FUNCTION "PALLET IMP.LAT. SU USCIT" : VOID
TITLE =GESTIONE PALLET PROVENIENTE DA IMPIL. LATERALE SU BAIA USCITA
VERSION : 0.1
//KNOW_HOW_PROTECT

VAR_TEMP
  Error_block_move : INT ;
END_VAR
BEGIN
NETWORK
TITLE =

NETWORK
TITLE =Spostamento dati per pallet in transito tra ribaltat. e uscita
//- "Container Flag"
//- "Id TAG"
//- "FlagRibaltamento"
//- "Container_Id"
//- "Date LCB"
//- "Part Number"
//- "Quantity"
//- "Line Id"
//- "CIM"
//- "Colata Id"
//- "Material Of Test Flag"
//- "Lotto Id"
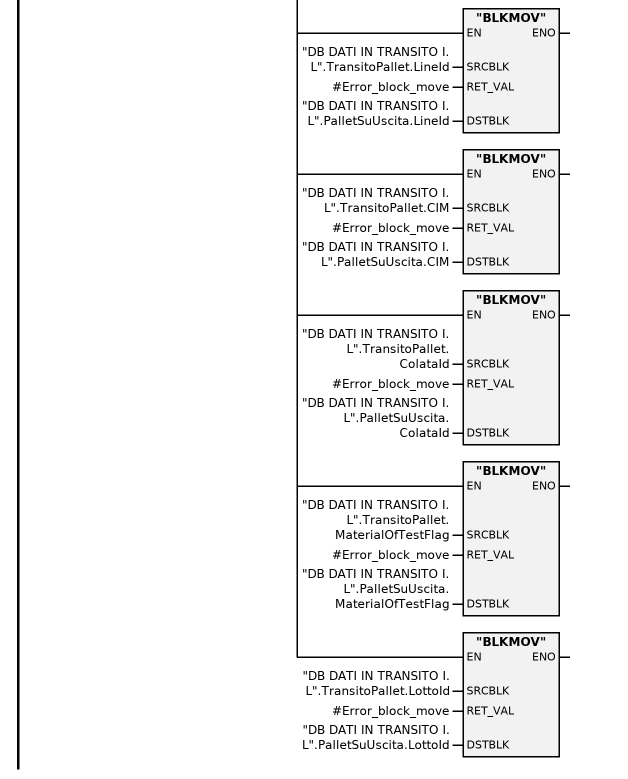
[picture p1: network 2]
      U     "M900.0";
      U     "DB SCAMBIO DATI PIANELLI".Pallet_I_L_su_uscita;
      FP    M    390.1;
      =     L      2.0;
      U     L      2.0;
      SPBNB _001;
      CALL "BLKMOV" (
           SRCBLK                   := "DB DATI IN TRANSITO I. L".TransitoPallet.ContainerFlag,
           RET_VAL                  := #Error_block_move,
           DSTBLK                   := "DB DATI IN TRANSITO I. L".PalletSuUscita.ContainerFlag);
_001: NOP   0;
      U     L      2.0;
      SPBNB _002;
      CALL "BLKMOV" (
           SRCBLK                   := "DB DATI IN TRANSITO I. L".TransitoPallet.ID_TAG,
           RET_VAL                  := #Error_block_move,
           DSTBLK                   := "DB DATI IN TRANSITO I. L".PalletSuUscita.ID_TAG);
_002: NOP   0;
      U     L      2.0;
      SPBNB _003;
      CALL "BLKMOV" (
           SRCBLK                   := "DB DATI IN TRANSITO I. L".TransitoPallet.FlagRibaltamento,
           RET_VAL                  := #Error_block_move,
           DSTBLK                   := "DB DATI IN TRANSITO I. L".PalletSuUscita.FlagRibaltamento);
_003: NOP   0;
      U     L      2.0;
      SPBNB _004;
      CALL "BLKMOV" (
           SRCBLK                   := "DB DATI IN TRANSITO I. L".TransitoPallet.Container_Id,
           RET_VAL                  := #Error_block_move,
           DSTBLK                   := "DB DATI IN TRANSITO I. L".PalletSuUscita.Container_Id);
_004: NOP   0;
      U     L      2.0;
      SPBNB _005;
      CALL "BLKMOV" (
           SRCBLK                   := "DB DATI IN TRANSITO I. L".TransitoPallet.DateLCB,
           RET_VAL                  := #Error_block_move,
           DSTBLK                   := "DB DATI IN TRANSITO I. L".PalletSuUscita.DateLCB);
_005: NOP   0;
      U     L      2.0;
      SPBNB _006;
      CALL "BLKMOV" (
           SRCBLK                   := "DB DATI IN TRANSITO I. L".TransitoPallet.PartNumber,
           RET_VAL                  := #Error_block_move,
           DSTBLK                   := "DB DATI IN TRANSITO I. L".PalletSuUscita.PartNumber);
_006: NOP   0;
      U     L      2.0;
      SPBNB _007;
      CALL "BLKMOV" (
           SRCBLK                   := "DB DATI IN TRANSITO I. L".TransitoPallet.Quantity,
           RET_VAL                  := #Error_block_move,
           DSTBLK                   := "DB DATI IN TRANSITO I. L".PalletSuUscita.Quantity);
_007: NOP   0;
      U     L      2.0;
      SPBNB _008;
      CALL "BLKMOV" (
           SRCBLK                   := "DB DATI IN TRANSITO I. L".TransitoPallet.LineId,
           RET_VAL                  := #Error_block_move,
           DSTBLK                   := "DB DATI IN TRANSITO I. L".PalletSuUscita.LineId);
_008: NOP   0;
      U     L      2.0;
      SPBNB _009;
      CALL "BLKMOV" (
           SRCBLK                   := "DB DATI IN TRANSITO I. L".TransitoPallet.CIM,
           RET_VAL                  := #Error_block_move,
           DSTBLK                   := "DB DATI IN TRANSITO I. L".PalletSuUscita.CIM);
_009: NOP   0;
      U     L      2.0;
      SPBNB _00a;
      CALL "BLKMOV" (
           SRCBLK                   := "DB DATI IN TRANSITO I. L".TransitoPallet.ColataId,
           RET_VAL                  := #Error_block_move,
           DSTBLK                   := "DB DATI IN TRANSITO I. L".PalletSuUscita.ColataId);
_00a: NOP   0;
      U     L      2.0;
      SPBNB _00b;
      CALL "BLKMOV" (
           SRCBLK                   := "DB DATI IN TRANSITO I. L".TransitoPallet.MaterialOfTestFlag,
           RET_VAL                  := #Error_block_move,
           DSTBLK                   := "DB DATI IN TRANSITO I. L".PalletSuUscita.MaterialOfTestFlag);
_00b: NOP   0;
      U     L      2.0;
      SPBNB _00c;
      CALL "BLKMOV" (
           SRCBLK                   := "DB DATI IN TRANSITO I. L".TransitoPallet.LottoId,
           RET_VAL                  := #Error_block_move,
           DSTBLK                   := "DB DATI IN TRANSITO I. L".PalletSuUscita.LottoId);
_00c: NOP   0;
NETWORK
TITLE =Lettura Pallet su baia di scarico
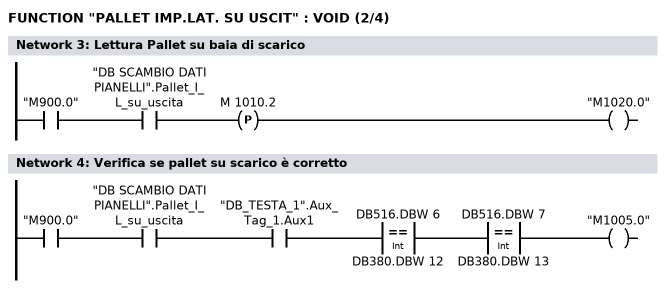
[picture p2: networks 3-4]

      U     "M900.0";
      U     "DB SCAMBIO DATI PIANELLI".Pallet_I_L_su_uscita;
      FP    M   1010.2;
      =     "M1020.0";
NETWORK
TITLE =Verifica se pallet su scarico è corretto

      U     "M900.0";
      U     "DB SCAMBIO DATI PIANELLI".Pallet_I_L_su_uscita;
      U     "DB_TESTA_1".Aux_Tag_1.Aux1;
      U(    ;
      L     DB516.DBW    6;
      L     DB380.DBW   12;
      ==I   ;
      )     ;
      U(    ;
      L     DB516.DBW    7;
      L     DB380.DBW   13;
      ==I   ;
      )     ;
      =     "M1005.0";
NETWORK
TITLE =Se pallet è corretto e ribaltato, aggiorno TAG
//- "Container Flag"
//- "Id TAG"
//- "FlagRibaltamento"
//- "Container_Id"
//- "Date LCB"
//- "Part Number"
//- "Quantity"
//- "Line Id"
//- "CIM"
//- "Colata Id"
//- "Material Of Test Flag"
//- "Lotto Id"
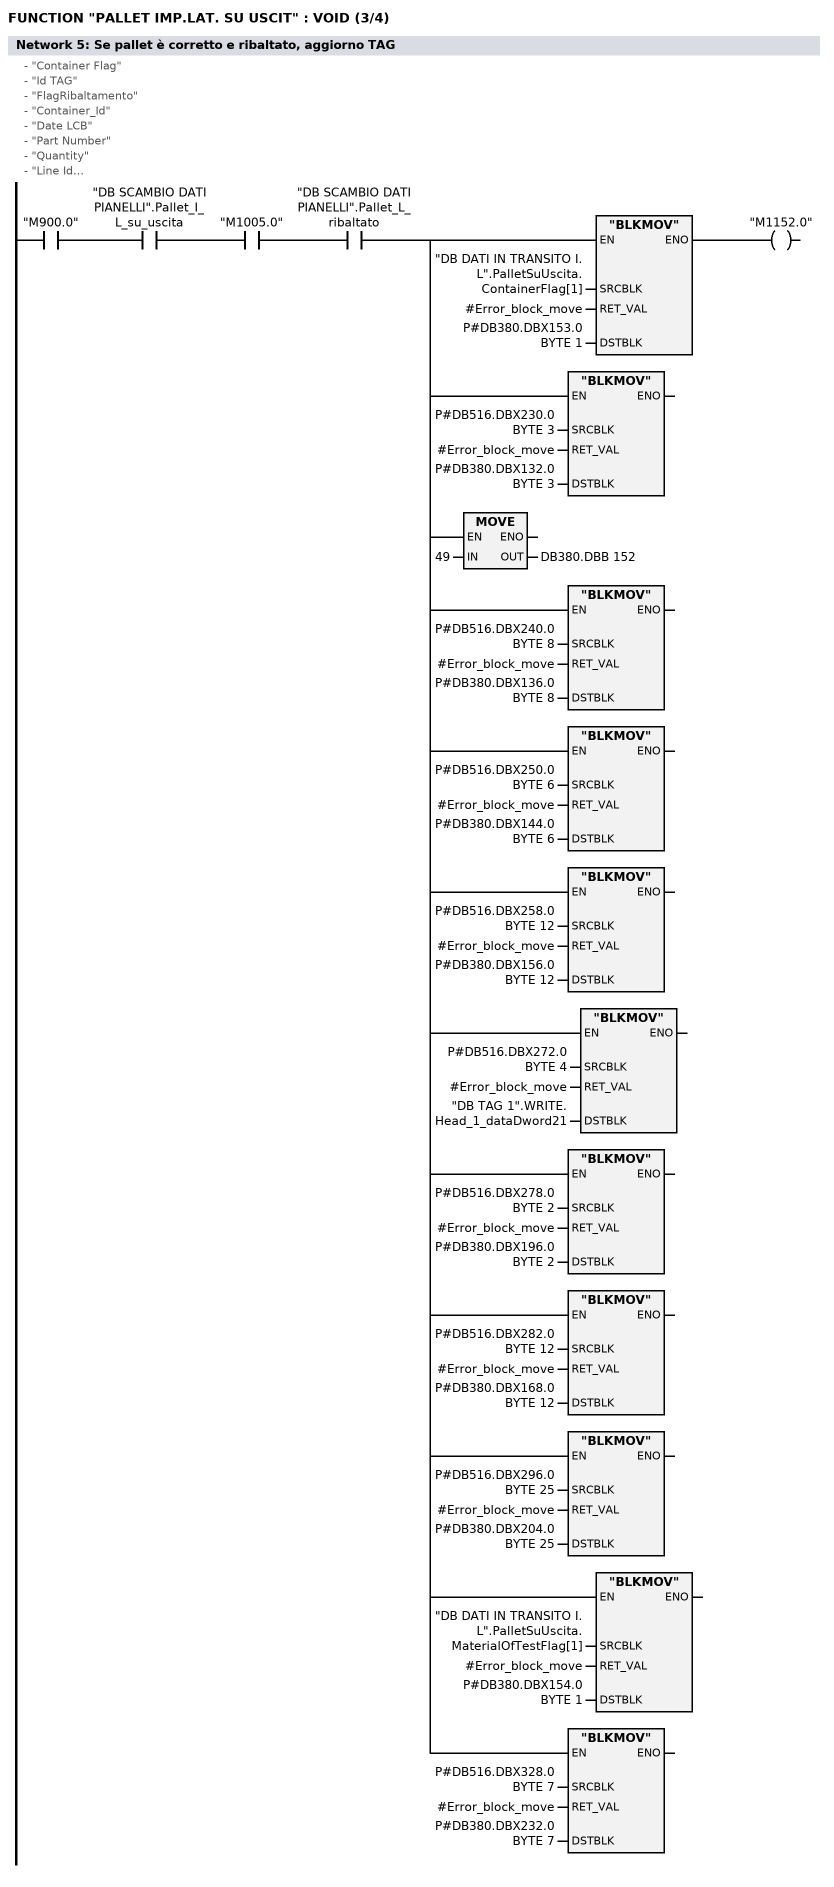
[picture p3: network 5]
      U     "M900.0";
      U     "DB SCAMBIO DATI PIANELLI".Pallet_I_L_su_uscita;
      U     "M1005.0";
      U     "DB SCAMBIO DATI PIANELLI".Pallet_L_ribaltato;
      =     L      2.0;
      U     L      2.0;
      SPBNB _00d;
      CALL "BLKMOV" (
           SRCBLK                   := "DB DATI IN TRANSITO I. L".PalletSuUscita.ContainerFlag[1],
           RET_VAL                  := #Error_block_move,
           DSTBLK                   := P#DB380.DBX153.0 BYTE 1);
_00d: U     BIE;
      =     "M1152.0";
      U     L      2.0;
      SPBNB _00e;
      CALL "BLKMOV" (
           SRCBLK                   := P#DB516.DBX230.0 BYTE 3,
           RET_VAL                  := #Error_block_move,
           DSTBLK                   := P#DB380.DBX132.0 BYTE 3);
_00e: NOP   0;
      U     L      2.0;
      SPBNB _00f;
      L     49;
      T     DB380.DBB  152;
_00f: NOP   0;
      U     L      2.0;
      SPBNB _010;
      CALL "BLKMOV" (
           SRCBLK                   := P#DB516.DBX240.0 BYTE 8,
           RET_VAL                  := #Error_block_move,
           DSTBLK                   := P#DB380.DBX136.0 BYTE 8);
_010: NOP   0;
      U     L      2.0;
      SPBNB _011;
      CALL "BLKMOV" (
           SRCBLK                   := P#DB516.DBX250.0 BYTE 6,
           RET_VAL                  := #Error_block_move,
           DSTBLK                   := P#DB380.DBX144.0 BYTE 6);
_011: NOP   0;
      U     L      2.0;
      SPBNB _012;
      CALL "BLKMOV" (
           SRCBLK                   := P#DB516.DBX258.0 BYTE 12,
           RET_VAL                  := #Error_block_move,
           DSTBLK                   := P#DB380.DBX156.0 BYTE 12);
_012: NOP   0;
      U     L      2.0;
      SPBNB _013;
      CALL "BLKMOV" (
           SRCBLK                   := P#DB516.DBX272.0 BYTE 4,
           RET_VAL                  := #Error_block_move,
           DSTBLK                   := "DB TAG 1".WRITE.Head_1_dataDword21);
_013: NOP   0;
      U     L      2.0;
      SPBNB _014;
      CALL "BLKMOV" (
           SRCBLK                   := P#DB516.DBX278.0 BYTE 2,
           RET_VAL                  := #Error_block_move,
           DSTBLK                   := P#DB380.DBX196.0 BYTE 2);
_014: NOP   0;
      U     L      2.0;
      SPBNB _015;
      CALL "BLKMOV" (
           SRCBLK                   := P#DB516.DBX282.0 BYTE 12,
           RET_VAL                  := #Error_block_move,
           DSTBLK                   := P#DB380.DBX168.0 BYTE 12);
_015: NOP   0;
      U     L      2.0;
      SPBNB _016;
      CALL "BLKMOV" (
           SRCBLK                   := P#DB516.DBX296.0 BYTE 25,
           RET_VAL                  := #Error_block_move,
           DSTBLK                   := P#DB380.DBX204.0 BYTE 25);
_016: NOP   0;
      U     L      2.0;
      SPBNB _017;
      CALL "BLKMOV" (
           SRCBLK                   := "DB DATI IN TRANSITO I. L".PalletSuUscita.MaterialOfTestFlag[1],
           RET_VAL                  := #Error_block_move,
           DSTBLK                   := P#DB380.DBX154.0 BYTE 1);
_017: NOP   0;
      U     L      2.0;
      SPBNB _018;
      CALL "BLKMOV" (
           SRCBLK                   := P#DB516.DBX328.0 BYTE 7,
           RET_VAL                  := #Error_block_move,
           DSTBLK                   := P#DB380.DBX232.0 BYTE 7);
_018: NOP   0;
NETWORK
TITLE =OK SCARICO PEDANA USCITA DA IMP_LATERALE
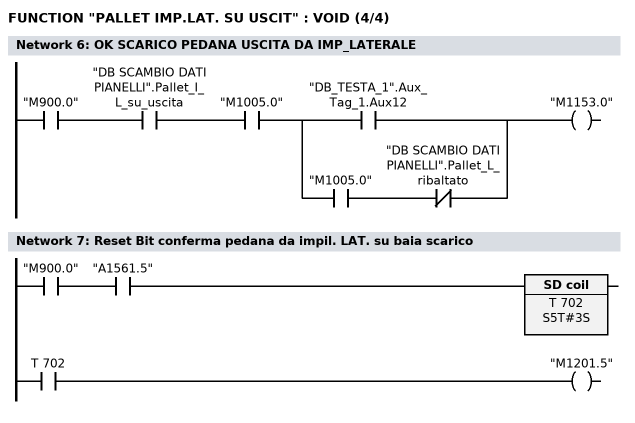
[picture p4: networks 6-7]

      U     "M900.0";
      U     "DB SCAMBIO DATI PIANELLI".Pallet_I_L_su_uscita;
      U     "M1005.0";
      U(    ;
      O     "DB_TESTA_1".Aux_Tag_1.Aux12;
      O     ;
      U     "M1005.0";
      UN    "DB SCAMBIO DATI PIANELLI".Pallet_L_ribaltato;
      )     ;
      =     "M1153.0";
NETWORK
TITLE =Reset Bit conferma pedana da impil. LAT. su baia scarico

      U     "M900.0";
      U     "A1561.5";
      L     S5T#3S;
      SE    T    702;
      NOP   0;
      NOP   0;
      NOP   0;
      U     T    702;
      =     "M1201.5";
END_FUNCTION

